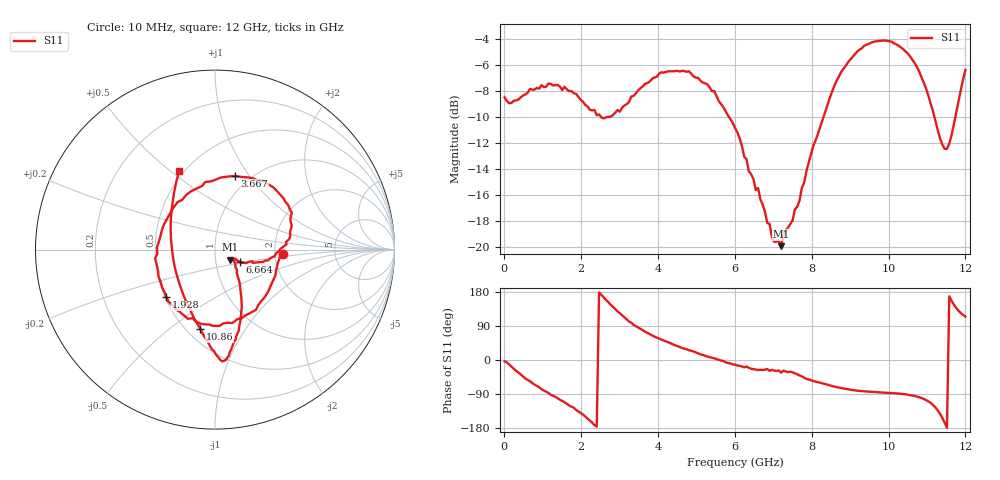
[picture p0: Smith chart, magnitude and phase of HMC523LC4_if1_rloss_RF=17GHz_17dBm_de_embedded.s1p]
!Hittite Microwave Corporation
!20 Alpha Rd
!Chelmsford, MA 01824
!Tel: 978-250-3343
!Fax: 978-250-3373
!Device: HMC523LC4, 0.01-12 GHz, GaAs MMIC Double-Balanced Mixer
!Misc: IF1 Return Loss with RF=17GHz at 17 dBm, Room
# MHZ S MA R 50
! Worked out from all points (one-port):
!   201 points, 10 MHz to 12 GHz, reference 50 ohm
!   lowest |S11| = -19.9 dB at 7.204 GHz (marker M1), VSWR 1.22, Z = 58.8 - j6.62 ohm
!   |S11| at or under -10 dB: 2.526 GHz to 2.661 GHz (135.3 MHz wide, 5.22 % of centre); 5.854 GHz to 8.306 GHz (2.453 GHz wide, 34.6 % of centre); 11.2 GHz to 11.74 GHz (540.5 MHz wide, 4.71 % of centre)
!   S11 on the Smith chart (normalised r, x): 10 MHz: 2.20, -0.12; 1.928 GHz: 0.51, -0.31; 3.667 GHz: 0.86, +0.86; 6.664 GHz: 1.31, -0.18; 10.86 GHz: 0.59, -0.65; 12 GHz: 0.47, +0.54
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10  0.377 -3.4
549.55  0.387 -49.0
849.3  0.41 -68.6
1149.05  0.426 -86.7
1508.75  0.402 -108.0
1928.4  0.379 -135.6
2467.95  0.324 177.9
3007.5  0.332 123.6
3307.25  0.38 98.4
3666.95  0.425 74.7
4086.6  0.471 54.0
4506.25  0.477 36.8
4806  0.475 25.7
5285.6  0.423 9.1
6005  0.288 -12.1
6664.45  0.153 -25.8
7024.15  0.105 -28.0
7204  0.101 -33.5
7503.75  0.127 -32.6
8522.9  0.394 -68.4
9002.5  0.526 -78.5
9781.85  0.622 -85.4
10501.25  0.556 -91.8
10860.95  0.449 -100.5
11160.7  0.332 -119.0
11400.5  0.248 -153.0
11520.4  0.239 -178.9
12000  0.48 114.6
